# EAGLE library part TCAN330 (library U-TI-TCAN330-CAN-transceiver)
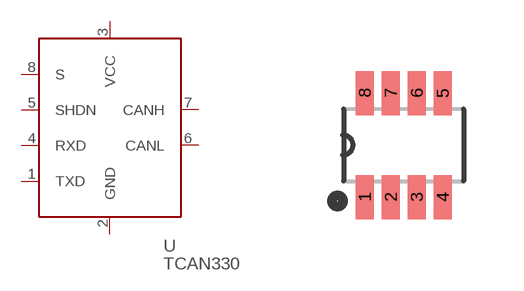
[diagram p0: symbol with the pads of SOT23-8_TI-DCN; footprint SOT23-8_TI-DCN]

Designator prefix U

## TCAN330  [SOT23-8_TI-DCN]
1  TXD  in
2  GND  pwr
3  VCC  pwr
4  RXD  out
5  SHDN  in
6  CANL
7  CANH
8  S  in

## Footprint SOT23-8_TI-DCN (pad centres in mm)
smd 0.45 x 1.1: 1 -0.975,-1.3; 2 -0.325,-1.3; 3 0.325,-1.3; 4 0.975,-1.3; 5 0.975,1.3; 6 0.325,1.3; 7 -0.325,1.3; 8 -0.975,1.3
